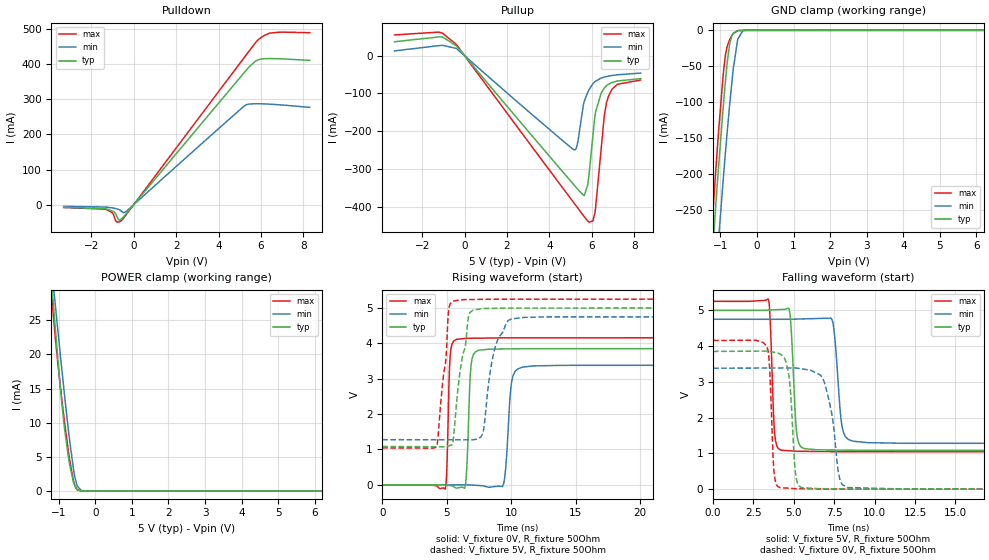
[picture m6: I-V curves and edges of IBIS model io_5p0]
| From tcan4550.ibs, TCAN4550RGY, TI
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|   io_5p0 Model
[Model]   io_5p0
Model_type   I/O
Polarity   Non-Inverting
Enable   Active-High
Vinl = 1.5
Vinh = 3.5
Vmeas = 2.5
Vref = 0
Cref = 2pF
Rref = 100000
|   typ   min   max
C_comp   9.071pF   7.937pF   9.499pF
|  Where Nom  PVT is Nominal Process, 5V,   27C
|   Fast PVT is Strong Process,  5.25, -40C
|   Slow PVT is Weak Process,   4.75V, 150C
[Model spec]
|subparameter
Vinl   1.5   1.425   1.575
Vinh   3.5   3.325   3.675
[Voltage Range]   5   4.75   5.25
|Junction Temperature
[Temperature Range]   27   150   -40
[Pullup Reference]   5   4.75   5.25
[Pulldown Reference]   0   0   0
[Power Clamp Reference]   5   4.75   5.25
[GND Clamp Reference]   0   0   0
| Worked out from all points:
|   slope of the pulldown table from 0 to 0.75 V, typ, clamps not added: 13.8 ohm
|   slope of the pullup table from 0 to 0.75 V, typ, clamps not added: 14.9 ohm
|   GND clamp passes 1 mA (typ) near -0.55 V on its own axis
|   POWER clamp passes 1 mA (typ) near -0.58 V on its own axis
|   falling waveform, V_fixture 5V, R_fixture 50Ohm: 20-80 % time 252ps typ, 345ps min, 200ps max; typ from 5 V to 1.08 V
|   rising waveform, V_fixture 0V, R_fixture 50Ohm: 20-80 % time 232ps typ, 346ps min, 180ps max; typ from 0 V to 3.85 V
|   rising waveform, V_fixture 5V, R_fixture 50Ohm: 20-80 % time 875ps typ, 919ps min, 614ps max; typ from 1.08 V to 5 V
|   falling waveform, V_fixture 0V, R_fixture 50Ohm: 20-80 % time 317ps typ, 640ps min, 218ps max; typ from 3.85 V to 0 V
[Pulldown]
|   Voltage   I(typ)   I(min)   I(max)
-3.3V     -7.557mA   -4.666mA   -7.918mA
-1.351V   -11.42mA   -6.665mA   -12.7mA
-1.015V   -17.81mA   -9.047mA   -22.63mA
-852.4mV  -25.33mA   -11.05mA   -46.16mA
-782.8mV  -33.8mA    -12.12mA   -49.72mA
-713.2mV  -42.39mA   -13.54mA   -49.32mA
-597.2mV  -41.69mA   -17.84mA   -46.09mA
-342mV    -24.78mA   -18.49mA   -27.55mA
5.191V    374.1mA    279.5mA    416.9mA
5.736V    408.1mA    287.2mA    460.4mA
6.398V    415.5mA    285.8mA    487.7mA
8.3V      410.4mA    276.8mA    489.1mA
[GND Clamp]
|   Voltage   I(typ)   I(min)   I(max)
-3.3V     -2.035A    -2.059A    -2.036A
-1.316V   -386.4mA   -483.2mA   -340mA
-1.131V   -247mA     -347.9mA   -198.4mA
-1.05V    -189.8mA   -291.5mA   -141mA
-922mV    -106.4mA   -207.4mA   -61.2mA
-875.6mV  -78.75mA   -178.6mA   -39.49mA
-748mV    -19.45mA   -104.5mA   -13.27mA
-643.6mV  -3.654mA   -52.25mA   -4.358mA
-527.6mV  -458.9uA   -12.72mA   -527.3uA
-388.4mV  -30.84uA   -654.5uA   -29.67uA
-295.6mV  -19.29uA   -75.02uA   -23.12uA
8.3V      0A         0A         0A
[Pullup]
|   Voltage   I(typ)   I(min)   I(max)
-3.3V     36.84mA    12.6mA     55.01mA
-1.212V   49.69mA    26.65mA    62.52mA
-388.4mV  26.1mA     19.23mA    29.6mA
5.18V     -343.9mA   -249.6mA   -392.1mA
5.33V     -353.8mA   -231.2mA   -403.4mA
5.644V    -370.6mA   -121mA     -426.9mA
5.899V    -298.5mA   -87.18mA   -441.4mA
6.177V    -148.9mA   -67.56mA   -402.9mA
6.583V    -86.03mA   -56.8mA    -161.2mA
6.769V    -76.33mA   -54.35mA   -110.4mA
7.21V     -67.17mA   -50.6mA    -75.84mA
8.3V      -60.75mA   -46.12mA   -64.52mA
[POWER Clamp]
|   Voltage   I(typ)   I(min)   I(max)
-3.3V     185.2mA    152.1mA    196.5mA
-1.2V     31.03mA    33.04mA    29.08mA
-1.189V   30.23mA    32.4mA     28.31mA
-1.177V   29.44mA    31.77mA    27.56mA
-1.096V   23.99mA    27.38mA    22.61mA
-945.2mV  14.56mA    19.38mA    14.83mA
-840.8mV  9.113mA    14.03mA    10.07mA
-701.6mV  3.868mA    7.389mA    4.535mA
-597.2mV  1.312mA    3.226mA    1.49mA
-492.8mV  192.3uA    712.2uA    165.6uA
-260.8mV  98.1nA     3.567uA    0A
8.3V      0A         0A         0A
[Ramp]
R_load = 50
|   typ   min   max
dV/dt_r   2.31072/2.31688e-10   2.02883/3.44752e-10   2.4944/1.77766e-10
dV/dt_f   2.35056/2.50666e-10   2.08315/3.44165e-10   2.52319/1.99421e-10
[Falling Waveform]
V_fixture = 5V
V_fixture_min = 4.75V
V_fixture_max = 5.25V
R_fixture = 50Ohm
C_fixture = 0F
|   Time   V(typ)   V(min)   V(max)
0s        5V         4.75V      5.25V
3.43ns    5.008V     4.75V      5.301V
3.807ns   5.015V     4.75V      1.589V
4.211ns   5.024V     4.75V      1.091V
4.757ns   4.921V     4.75V      1.073V
5.174ns   1.584V     4.755V     1.06V
5.655ns   1.133V     4.761V     1.057V
7.34ns    1.096V     4.761V     1.05V
8.649ns   1.088V     1.344V     1.048V
33ns      1.082V     1.278V     1.045V
[Rising Waveform]
V_fixture = 0V
V_fixture_min = 0V
V_fixture_max = 0V
R_fixture = 50Ohm
C_fixture = 0F
|   Time   V(typ)   V(min)   V(max)
0s        177.2uV    204.4uV    198.5uV
4.883ns   -3.992mV   406.6uV    -121.5mV
5.256ns   -19.36mV   422uV      3.592V
5.744ns   -93.18mV   442.2uV    4.11V
6.454ns   8.075mV    471.6uV    4.136V
6.878ns   3.36V      -2.423mV   4.143V
7.447ns   3.8V       -17.07mV   4.145V
9.333ns   3.84V      -39.05mV   4.154V
10.81ns   3.847V     3.321V     4.154V
33ns      3.851V     3.382V     4.158V
[Rising Waveform]
V_fixture = 5V
V_fixture_min = 4.75V
V_fixture_max = 5.25V
R_fixture = 50Ohm
C_fixture = 0F
|   Time   V(typ)   V(min)   V(max)
0s        1.082V     1.278V     1.045V
4.22ns    1.077V     1.275V     1.09V
5.141ns   1.098V     1.274V     4.901V
5.492ns   1.247V     1.274V     5.193V
6.102ns   3.382V     1.274V     5.229V
7.038ns   4.94V      1.274V     5.238V
7.786ns   4.981V     1.445V     5.242V
8.685ns   4.989V     3.799V     5.246V
9.998ns   4.995V     4.686V     5.246V
33ns      5V         4.75V      5.25V
[Falling Waveform]
|Gnd
V_fixture = 0V
V_fixture_min = 0V
V_fixture_max = 0V
R_fixture = 50Ohm
C_fixture = 0F
|   Time   V(typ)   V(min)   V(max)
0s        3.851V     3.382V     4.158V
3.341ns   3.86V      3.387V     3.96V
3.774ns   3.827V     3.388V     495.6mV
4.132ns   3.781V     3.388V     43.11mV
4.702ns   3.154V     3.389V     26.42mV
5.115ns   396mV      3.389V     14.8mV
5.503ns   43.89mV    3.363V     12.71mV
6.796ns   13.47mV    3.096V     7.801mV
8.295ns   7.322mV    47.76mV    3.68mV
33ns      177.3uV    204.5uV    198.5uV
